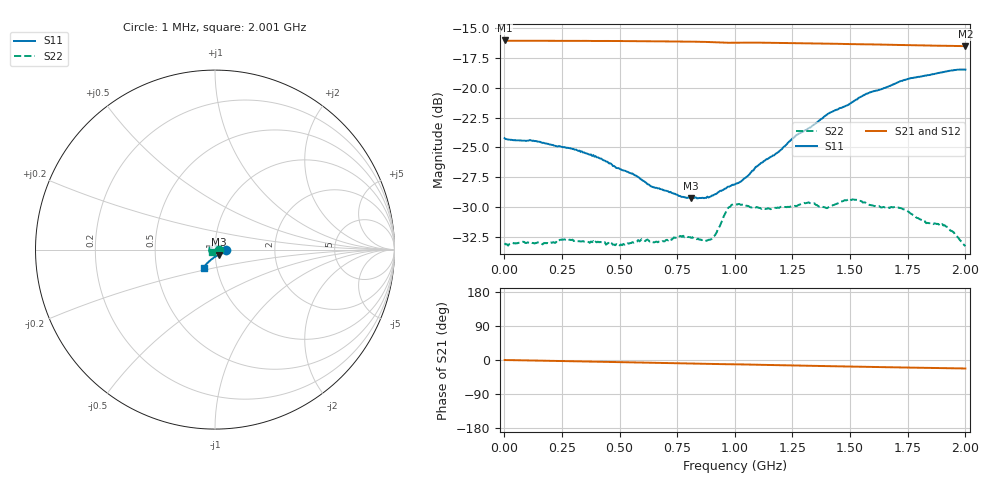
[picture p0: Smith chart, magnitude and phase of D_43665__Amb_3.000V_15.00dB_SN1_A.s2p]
! device id: 43665_
! dir: \\malibu\benchdata\1_engineers\tn_data\43665_75ohm\new\sparar\43665_\amb\3p000v\15p00db
! Serial: 1
! Insertion: A
! Temp: Amb
! VDD: 3.000V
! Attenuation Step: 15.00dB
! IDD: 1.444926e+00mA
! FILE NAME
! DATE 03-27-2009 08:37:02
! CORRECTED  DATA
#  Hz  S  RI  R  75
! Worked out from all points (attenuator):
!   401 points, 1 MHz to 2.001 GHz, reference 75 ohm
!   highest |S21| = -16.06 dB at 1 MHz (marker M1); lowest = -16.5 dB at 2.001 GHz (marker M2)
!   lowest |S11| = -29.2 dB at 811 MHz (marker M3), VSWR 1.07, Z = 77.9 - j4.43 ohm
!   |S11| at or under -10 dB: start of sweep to end of sweep
!   |S22| runs from -33.2 to -29.3 dB; largest |S21 - S12| = 0.00043
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1000000  0.0615 -0.000692  0.1573 -0.000352  0.1571 -0.000254  0.0224 -0.000195
1.36e8  0.0597 -0.00326  0.1568 -0.00408  0.1569 -0.00404  0.0208 0.0085
2.66e8  0.0557 -0.00713  0.1566 -0.00807  0.1566 -0.00808  0.0174 0.0154
3.36e8  0.0535 -0.00901  0.1564 -0.0102  0.1564 -0.0102  0.0135 0.0184
5.01e8  0.0435 -0.0143  0.1556 -0.0154  0.1557 -0.0154  0.00476 0.0214
5.91e8  0.0375 -0.0178  0.155 -0.0181  0.155 -0.0181  -0.00186 0.0229
6.71e8  0.0311 -0.0218  0.1546 -0.0206  0.1546 -0.0205  -0.00572 0.022
8.11e8  0.0196 -0.0284  0.1534 -0.0251  0.1535 -0.0251  -0.0146 0.0185
8.71e8  0.0141 -0.0316  0.1527 -0.0272  0.1527 -0.0271  -0.0177 0.0145
9.01e8  0.0109 -0.0337  0.1522 -0.0282  0.1522 -0.0281  -0.0198 0.0124
9.26e8  0.00827 -0.0355  0.1516 -0.0289  0.1517 -0.0287  -0.0229 0.0112
9.66e8  0.00525 -0.0379  0.1511 -0.0294  0.1511 -0.0293  -0.0285 0.0119
1.001e9  0.00193 -0.0394  0.151 -0.0302  0.1511 -0.03  -0.0299 0.0131
1.146e9  -0.012 -0.0492  0.1498 -0.0349  0.1499 -0.0347  -0.0305 0.00723
1.336e9  -0.0295 -0.0626  0.1475 -0.0403  0.1478 -0.0402  -0.0328 -0.00266
1.401e9  -0.0354 -0.0686  0.1467 -0.0424  0.147 -0.0424  -0.0308 -0.00602
1.521e9  -0.0446 -0.0762  0.1448 -0.0455  0.1452 -0.0455  -0.0324 -0.0103
1.671e9  -0.0535 -0.0863  0.1427 -0.0494  0.1428 -0.0495  -0.0289 -0.0123
1.736e9  -0.0571 -0.0912  0.1416 -0.051  0.1419 -0.0512  -0.0274 -0.0145
1.831e9  -0.0594 -0.0952  0.1402 -0.0531  0.1401 -0.0534  -0.0237 -0.0132
1.911e9  -0.0629 -0.098  0.1391 -0.0549  0.1391 -0.0549  -0.0231 -0.0133
2.001e9  -0.0637 -0.1003  0.1377 -0.0567  0.1376 -0.0571  -0.0186 -0.0113
